FUNCTION_BLOCK FB_PositionSource
VAR_INPUT
	t : LREAL;
	rpm: LREAL;
END_VAR
VAR_OUTPUT
	pos : LREAL;
END_VAR
VAR
	m_lasttime : LREAL;
	m_lastpos : LREAL;
	m_actpos : LREAL;
m_diff_t : LREAL;	
END_VAR

m_diff_t := (t - m_lasttime);
pos := m_lastpos + m_diff_t * rpm / 60.0;
m_lastpos := pos;
m_lasttime := t;

END_FUNCTION_BLOCK
